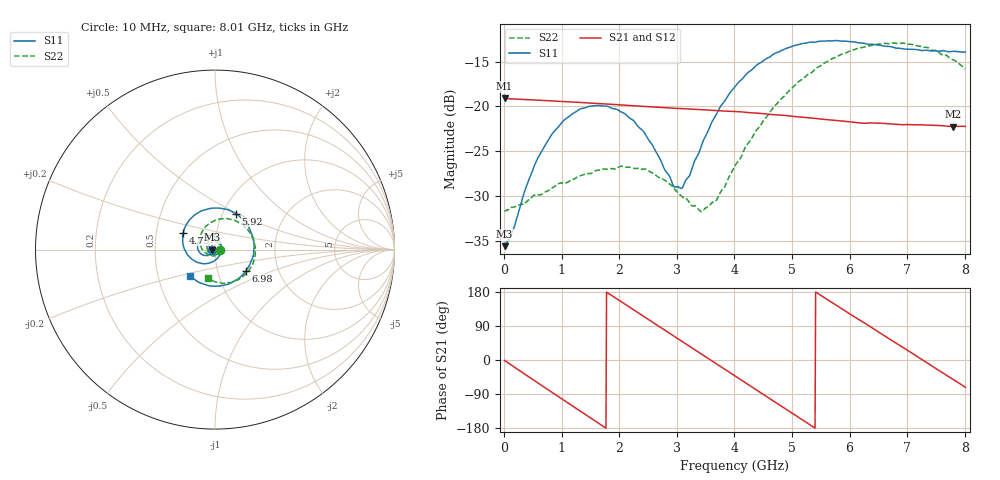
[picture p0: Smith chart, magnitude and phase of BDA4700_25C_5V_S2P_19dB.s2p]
!Agilent Technologies,E5071B,MY42404982,A.09.10
!Date: Mon Oct 20 13:35:51 2025
!Data & Calibration Information:
!Freq	S11:SOLT2(ON)	S21:SOLT2(ON)	S12:SOLT2(ON)	S22:SOLT2(ON)
# Hz S RI R 50
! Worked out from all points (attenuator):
!   801 points, 10 MHz to 8.01 GHz, reference 50 ohm
!   highest |S21| = -19.09 dB at 10 MHz (marker M1); lowest = -22.2 dB at 7.8 GHz (marker M2)
!   lowest |S11| = -35.6 dB at 10 MHz (marker M3), VSWR 1.03, Z = 48.4 - j0.11 ohm
!   |S11| at or under -10 dB: start of sweep to end of sweep
!   |S22| runs from -31.7 to -12.9 dB; largest |S21 - S12| = 0.00088
!   S11 on the Smith chart (normalised r, x): 10 MHz: 0.97, -0.00; 4.75 GHz: 0.69, +0.14; 5.92 GHz: 1.15, +0.49; 6.98 GHz: 1.37, -0.34; 8.01 GHz: 0.73, -0.22
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1e7  -0.0166 -0.00113  0.111 -0.00241  0.111 -0.00249  0.0262 -0.000879
1.5e8  -0.0178 -0.0096  0.1059 -0.0299  0.106 -0.0299  0.0264 -0.00729
3.9e8  -0.0266 -0.0245  0.0832 -0.0707  0.0832 -0.0708  0.0209 -0.0207
6.3e8  -0.0433 -0.033  0.0461 -0.0979  0.0461 -0.098  0.0103 -0.0304
1.02e9  -0.0792 -0.0229  -0.0264 -0.1033  -0.0265 -0.1033  -0.0173 -0.0331
1.35e9  -0.0972 0.00818  -0.0777 -0.0709  -0.0778 -0.0709  -0.0378 -0.0166
2.08e9  -0.0481 0.0783  -0.0873 0.0523  -0.0874 0.0523  -0.0278 0.0366
2.42e9  -0.00203 0.0727  -0.0427 0.0906  -0.0427 0.0907  -0.00103 0.0447
2.68e9  0.0251 0.0466  0.000955 0.0991  0.00089 0.0991  0.0172 0.0365
2.94e9  0.035 0.00907  0.0433 0.0877  0.0433 0.0876  0.0285 0.0209
3.09e9  0.0319 -0.0145  0.064 0.0732  0.0637 0.0734  0.0304 0.00831
3.46e9  -0.00584 -0.0643  0.0937 0.0205  0.0937 0.0205  0.0169 -0.0204
3.69e9  -0.0471 -0.0775  0.0933 -0.017  0.0933 -0.0172  -0.00219 -0.0299
4.01e9  -0.1116 -0.0643  0.0696 -0.0627  0.0696 -0.0626  -0.0369 -0.0282
4.75e9  -0.177 0.0944  -0.0385 -0.0809  -0.0384 -0.0811  -0.0833 0.0632
5.35e9  -0.0631 0.2197  -0.0857 -0.00788  -0.0858 -0.00814  -0.0136 0.1551
5.92e9  0.1154 0.2008  -0.0527 0.0637  -0.0529 0.0635  0.12 0.1582
6.68e9  0.2149 -0.0232  0.044 0.0669  0.0442 0.0668  0.2241 -0.00886
6.98e9  0.1727 -0.1175  0.07 0.0372  0.07 0.0369  0.2043 -0.0903
7.39e9  0.0564 -0.1969  0.077 -0.0161  0.077 -0.0163  0.1234 -0.1698
7.8e9  -0.0838 -0.185  0.0482 -0.0604  0.048 -0.0607  0.00907 -0.1817
8.01e9  -0.1408 -0.1443  0.0238 -0.0737  0.024 -0.0737  -0.0407 -0.157
